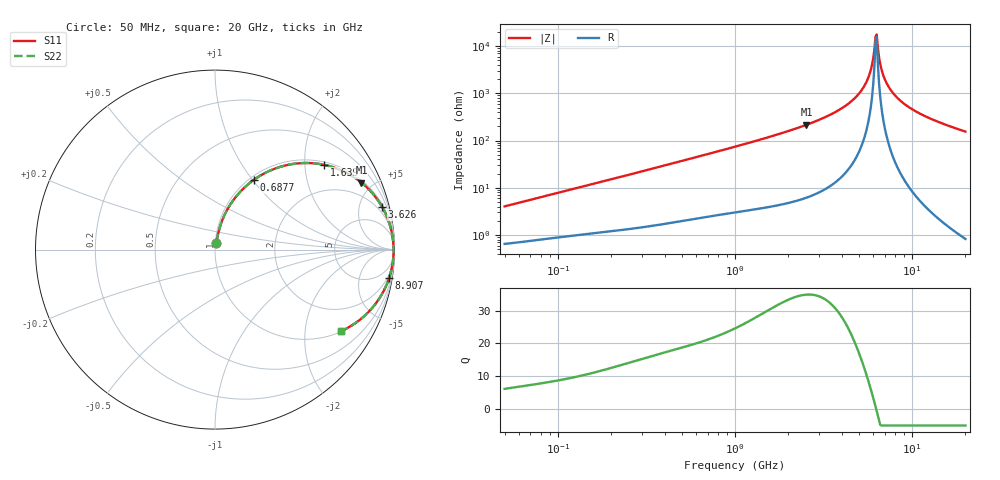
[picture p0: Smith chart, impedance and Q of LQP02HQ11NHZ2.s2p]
!Murata Part Number: LQP02HQ11NHZ2
!These Parameters are Measured in Series Mode Connection
!  o--[Z]--o
!Port1  Port2
!  o-------o
!Freq. Start=50[MHz] Stop=20[GHz], 401[Steps]
# Hz S RI R 50
!Freq.(Hz) S11(Real) S11(Imag) S21(Real) S21(Imag) S12(Real) S12(Imag) S22(Real) S22(Imag)
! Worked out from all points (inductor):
!   401 points, 50 MHz to 20 GHz, reference 50 ohm
!   read as one part in series: L = 12.6 nH near 51.52 MHz
!   highest Q = 34.9 at 2.531 GHz (marker M1), where L = 13.5 nH
!   self-resonance near 6.218 GHz
!   S11 on the Smith chart (normalised r, x): 50 MHz: 1.01, +0.08; 687.7 MHz: 1.05, +1.01; 1.639 GHz: 1.08, +2.51; 3.626 GHz: 1.25, +7.74; 8.907 GHz: 1, -12; 20 GHz: 1.02, -3.10
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5e7  0.008 0.0393  0.992 -0.0393  0.992 -0.0393  0.008 0.0393
1.364002e8  0.0205 0.1009  0.9795 -0.1009  0.9795 -0.1009  0.0205 0.1009
3.721004e8  0.0838 0.2488  0.9162 -0.2488  0.9162 -0.2488  0.0838 0.2488
6.87656e8  0.2152 0.3879  0.7848 -0.3879  0.7848 -0.3879  0.2152 0.3879
1e9  0.3593 0.4599  0.6407 -0.4599  0.6407 -0.4599  0.3593 0.4599
1.639343e9  0.6093 0.472  0.3907 -0.472  0.3907 -0.472  0.6093 0.472
2.531158e9  0.8156 0.3738  0.1844 -0.3738  0.1844 -0.3738  0.8156 0.3738
2.728004e9  0.8444 0.3484  0.1556 -0.3484  0.1556 -0.3484  0.8444 0.3484
3.626126e9  0.9307 0.2384  0.0693 -0.2384  0.0693 -0.2384  0.9307 0.2384
4.539627e9  0.9726 0.1427  0.0274 -0.1427  0.0274 -0.1427  0.9726 0.1427
5.273168e9  0.9884 0.0769  0.0116 -0.0769  0.0116 -0.0769  0.9884 0.0769
5.769027e9  0.9933 0.0372  0.00666 -0.0372  0.00666 -0.0372  0.9933 0.0372
5.944466e9  0.9943 0.0239  0.00573 -0.0239  0.00573 -0.0239  0.9943 0.0239
6.125241e9  0.9948 0.0106  0.00516 -0.0106  0.00516 -0.0106  0.9948 0.0106
6.217679e9  0.995 0.00391  0.00501 -0.00391  0.00501 -0.00391  0.995 0.00391
6.406762e9  0.995 -0.00941  0.00498 0.00941  0.00498 0.00941  0.995 -0.00941
6.701223e9  0.9944 -0.0294  0.00562 0.0294  0.00562 0.0294  0.9944 -0.0294
6.905011e9  0.9935 -0.0427  0.00651 0.0427  0.00651 0.0427  0.9935 -0.0427
7.442007e9  0.9897 -0.076  0.0103 0.076  0.0103 0.076  0.9897 -0.076
8.907419e9  0.971 -0.1555  0.029 0.1555  0.029 0.1555  0.971 -0.1555
1.238412e10  0.8993 -0.2954  0.1007 0.2954  0.1007 0.2954  0.8993 -0.2954
2e10  0.7047 -0.4535  0.2953 0.4535  0.2953 0.4535  0.7047 -0.4535
